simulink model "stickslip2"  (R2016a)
settings: Solver=ode45  SolverMode=SingleTasking  StartTime=0.0  StopTime=10  FixedStep=0.001  MaxStep=0.01  RelTol=1e-3  AbsTol=1e-6
InitFcn:
  | m = 1;
undefined symbols (not defined in the file or in its folder): FN, mug, muh, v0

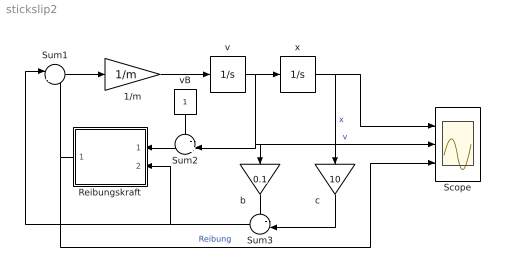
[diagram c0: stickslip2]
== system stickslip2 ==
  1/m : Gain  Gain=1/m
  Reibungskraft : Subsystem
  Scope : Scope  NumInputPorts=3
  Sum1 : Sum  Inputs=|++
  Sum2 : Sum  Inputs=-+|
  Sum3 : Sum  Inputs=--|
  b : Gain  Gain=0.1
  c : Gain  Gain=10
  v : Integrator
  vB : Constant
  x : Integrator  UpperSaturationLimit=100  LowerSaturationLimit=-100
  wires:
  x/1 -> Scope/1, c/1  "x"
  Sum1/1 -> 1/m/1
  v/1 -> x/1, Sum2/2, b/1, Scope/2  "v"
  1/m/1 -> v/1
  Reibungskraft/1(FR) -> Scope/3, Sum1/2  "Reibung"
  Sum3/1 -> Sum1/1, Reibungskraft/2(Fext)
  Sum2/1 -> Reibungskraft/1(v)
  vB/1 -> Sum2/1
  b/1 -> Sum3/1
  c/1 -> Sum3/2

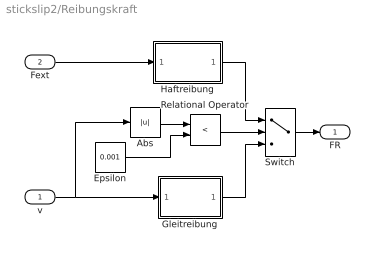
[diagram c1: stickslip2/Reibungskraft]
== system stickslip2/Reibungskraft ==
  v : Inport
  Fext : Inport  Port=2
  Abs : Abs
  Epsilon : Constant  Value=0.001
  Gleitreibung : Subsystem
  Haftreibung : Subsystem
  Relational Operator : RelationalOperator  Operator=<
  Switch : Switch  Threshold=0.5
  FR : Outport
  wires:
  Fext/1 -> Haftreibung/1(Fext)
  Relational Operator/1 -> Switch/2
  Gleitreibung/1(Fg) -> Switch/3
  Haftreibung/1(Fh) -> Switch/1
  Epsilon/1 -> Relational Operator/2
  Abs/1 -> Relational Operator/1
  v/1 -> Abs/1, Gleitreibung/1(v)
  Switch/1 -> FR/1

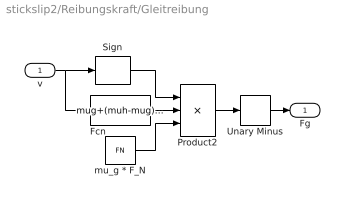
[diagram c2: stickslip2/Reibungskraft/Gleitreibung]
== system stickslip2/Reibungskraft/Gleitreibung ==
  v : Inport
  Fcn : Fcn  Expr=mug+(muh-mug)*exp(-abs(u)/v0)
  Product2 : Product  Inputs=3
  Sign : Signum
  Unary Minus : UnaryMinus
  mu_g * F_N : Constant  Value=FN
  Fg : Outport
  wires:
  mu_g * F_N/1 -> Product2/3
  Fcn/1 -> Product2/2
  Unary Minus/1 -> Fg/1
  Product2/1 -> Unary Minus/1
  v/1 -> Fcn/1, Sign/1
  Sign/1 -> Product2/1

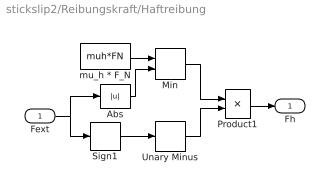
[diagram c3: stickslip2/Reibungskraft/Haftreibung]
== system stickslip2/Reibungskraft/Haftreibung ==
  Fext : Inport
  Abs : Abs
  Min : MinMax  Inputs=2
  Product1 : Product
  Sign1 : Signum
  Unary Minus : UnaryMinus
  mu_h * F_N : Constant  Value=muh*FN
  Fh : Outport
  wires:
  Abs/1 -> Min/2
  mu_h * F_N/1 -> Min/1
  Min/1 -> Product1/1
  Fext/1 -> Sign1/1, Abs/1
  Product1/1 -> Fh/1
  Sign1/1 -> Unary Minus/1
  Unary Minus/1 -> Product1/2
